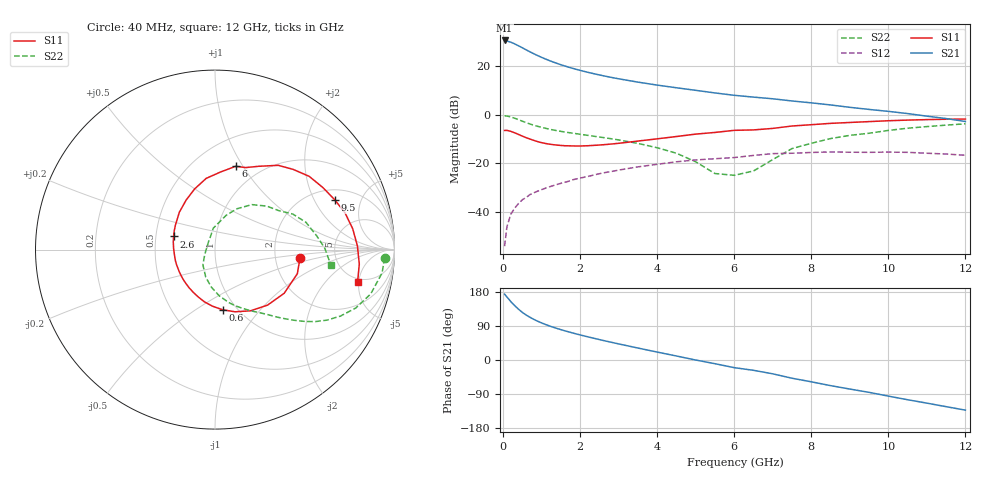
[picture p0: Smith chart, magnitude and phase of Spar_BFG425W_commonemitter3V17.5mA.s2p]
! Filename: 317bfg425.001
! BFG425W Field C1
! V1=8.486E-001V,V2=3.000E+000V, I1=2.294E-004A, I2=1.752E-002A
# GHz  S  MA  R 50
!  S11  S21  S12  S22
!Freq(GHz)  Mag  Ang  Mag  Ang  Mag  Ang  Mag  Ang
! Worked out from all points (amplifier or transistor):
!   44 points, 40 MHz to 12 GHz, reference 50 ohm
!   highest |S21| = 30.5 dB at 40 MHz (marker M1)
!   |S21| within 3 dB of that: start of sweep to 499.2 MHz
!   unconditionally stable (mu >= 1): 1.45 GHz to end of sweep
!   at 700 MHz: K = 0.70, MSG = 29.3 dB, |S12| = -32.8 dB
!   at 2.4 GHz: K = 1.14, MAG = 18.4 dB, |S12| = -24.6 dB
!   at 12 GHz: K = 1.35, MAG = 3.4 dB, |S12| = -16.7 dB
!   S11 on the Smith chart (normalised r, x): 40 MHz: 2.77, -0.34; 600 MHz: 0.86, -0.65; 2.6 GHz: 0.62, +0.10; 6 GHz: 0.77, +0.93; 9.5 GHz: 2.55, +2.96; 12 GHz: 4.44, -4.83
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0.04  0.476 -5.7  33.52 173.7  0.002 67.0  0.946 -2.8
0.1  0.478 -16.4  32.63 166.4  0.005 81.5  0.94 -8.0
0.2  0.456 -32.2  30.89 154.2  0.009 75.7  0.902 -15.9
0.3  0.426 -46.5  28.57 143.6  0.012 71.3  0.849 -22.6
0.4  0.394 -60.0  26.09 134.1  0.015 67.9  0.791 -27.9
0.5  0.364 -72.1  23.71 125.6  0.018 64.5  0.737 -32.2
0.6  0.338 -82.7  21.49 118.6  0.02 62.5  0.688 -35.7
0.7  0.316 -92.4  19.54 112.6  0.023 60.7  0.645 -38.4
0.9  0.28 -109.5  16.36 102.2  0.027 58.7  0.577 -42.7
1  0.267 -117.0  15.07 97.8  0.029 57.9  0.55 -44.5
1.2  0.249 -130.6  12.96 90.0  0.033 56.6  0.506 -47.8
1.6  0.231 -154.0  10.04 77.1  0.041 54.0  0.442 -53.4
2.2  0.231 178.0  7.436 61.1  0.054 48.9  0.377 -62.3
2.6  0.242 162.3  6.314 51.5  0.064 44.7  0.34 -68.7
3.5  0.288 133.6  4.676 31.6  0.085 33.5  0.258 -84.9
4.5  0.357 108.4  3.578 10.6  0.108 19.1  0.162 -108.5
6  0.478 76.1  2.507 -20.2  0.132 -5.3  0.057 128.9
6.5  0.488 69.5  2.301 -27.2  0.146 -8.4  0.07 113.8
8.5  0.665 37.8  1.589 -67.6  0.172 -45.4  0.324 50.7
9.5  0.723 22.5  1.285 -85.3  0.169 -62.1  0.417 31.3
10.5  0.776 8.6  1.057 -104.8  0.169 -80.8  0.529 16.7
12  0.815 -13.0  0.726 -132.3  0.147 -110.8  0.651 -7.6
